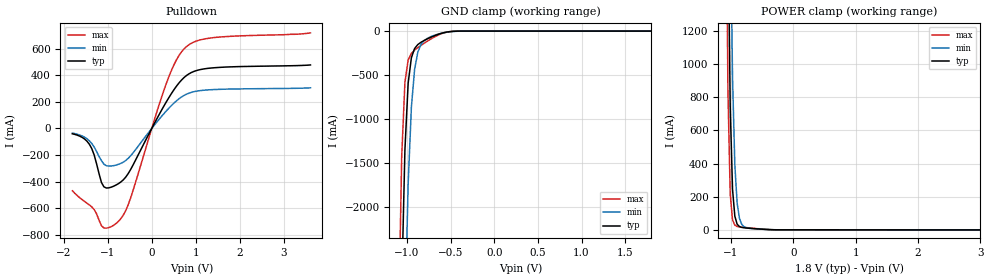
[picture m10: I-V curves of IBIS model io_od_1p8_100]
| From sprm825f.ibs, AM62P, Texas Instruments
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|   Model io_od_1p8_100
[Model]   io_od_1p8_100
Model_type   I/O_open_drain
Polarity   Non-Inverting
Enable   Active-High
Vinl =  0.630V
Vinh =  1.170V
Vmeas = 0.900V
Cref =  50.000pF
Rref =  4.700k
Vref =  1.800V
|   typ   min   max
C_comp   8.019pF   6.288pF   10.308pF
[Model Spec]
Vinh   1.170V   1.053V   1.287V
Vinl   0.630V   0.567V   0.693V
[Voltage Range]   1.8   1.62   1.98
[Temperature Range]   30   125   -40
[Pullup Reference]   1.8   1.62   1.98
[Pulldown Reference]   0   0   0
[Power Clamp Reference]   1.8   1.62   1.98
[GND Clamp Reference]   0   0   0
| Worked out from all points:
|   slope of the pulldown table from 0 to 0.27 V, typ, clamps not added: 1.64 ohm
|   GND clamp passes 1 mA (typ) near -0.43 V on its own axis
|   POWER clamp passes 1 mA (typ) near -0.37 V on its own axis
[Pulldown]
|Voltage   I(typ)   I(min)   I(max)
-1.8V     -39.91mA   -34.99mA   -468.3mA
-1.415V   -118.2mA   -92.43mA   -574.3mA
-1.305V   -199.6mA   -139.7mA   -609.7mA
-1.14V    -405.9mA   -241.7mA   -730.7mA
-1.085V   -438.4mA   -268.3mA   -747.8mA
-700mV    -402mA     -262.4mA   -677.5mA
-480mV    -309.3mA   -205.8mA   -523.4mA
400mV     238mA      156.5mA    398.7mA
620mV     342.9mA    223.5mA    549.2mA
840mV     409.6mA    264.9mA    628.5mA
1.445V    457mA      292.9mA    684.2mA
3.6V      477.3mA    305.5mA    718.3mA
[GND_clamp]
|Voltage   I(typ)   I(min)   I(max)
-1.8V     -76.47A    -76.69A    -88.72A
-1.097V   -5.386A    -8.269A    -3.42A
-1.06V    -2.917A    -5.464A    -1.424A
-1.023V   -1.346A    -3.251A    -578.9mA
-986mV    -591.1mA   -1.735A    -328.6mA
-949mV    -302.3mA   -863.2mA   -252.5mA
-912mV    -197.4mA   -432.7mA   -215.7mA
-875mV    -152.6mA   -237.8mA   -187.7mA
-838mV    -126.3mA   -149.6mA   -161.9mA
-727mV    -70.56mA   -63.46mA   -90.7mA
-468mV    -2.661mA   -4.447mA   -1.949mA
1.8V      0A         0A         0A
[POWER_clamp]
|Voltage   I(typ)   I(min)   I(max)
-1.8V     48.67A     48.99A     48.49A
-1.086V   4.074A     6.144A     2.54A
-1.049V   1.948A     3.749A     845.8mA
-1.012V   740.1mA    1.988A     214.2mA
-975mV    244.4mA    922.4mA    60.18mA
-938mV    82.37mA    391.6mA    27.84mA
-901mV    33.98mA    161.7mA    20.41mA
-864mV    19.43mA    69.17mA    17.82mA
-827mV    14.52mA    32.82mA    16.17mA
-753mV    10.9mA     12.35mA    13.31mA
-272mV    149.6uA    291uA      119.3uA
3.6V      -838.1uA   -712.3uA   -1.009mA
[Ramp]
| variable   typ   min   max
dV/dt_r   1.047/0.322n   0.927/0.372n   1.166/0.302n
dV/dt_f   1.047/91.572p   0.927/0.143n   1.166/62.513p
R_load = 50.000
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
